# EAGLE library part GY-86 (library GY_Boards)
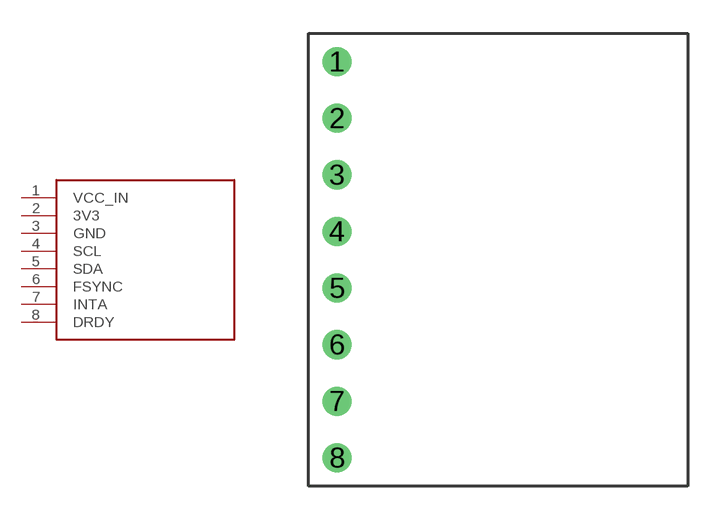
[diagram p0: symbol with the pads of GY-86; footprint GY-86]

Designator prefix -

## GY-86  [GY-86]
1  VCC_IN  oc
2  3V3  out
3  GND  pwr
4  SCL  nc
5  SDA
6  FSYNC
7  INTA
8  DRDY  out

## Footprint GY-86 (pad centres in mm)
drill 0.8: 1 1.27,19.05; 2 1.27,16.51; 3 1.27,13.97; 4 1.27,11.43; 5 1.27,8.89; 6 1.27,6.35; 7 1.27,3.81; 8 1.27,1.27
